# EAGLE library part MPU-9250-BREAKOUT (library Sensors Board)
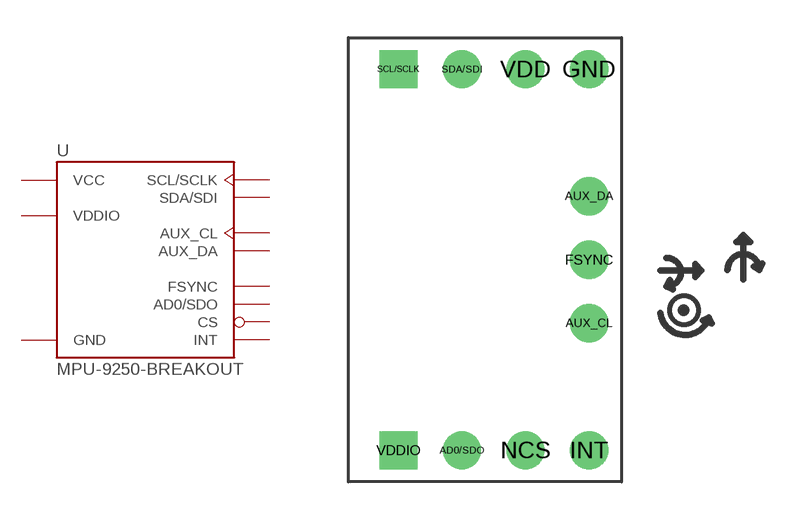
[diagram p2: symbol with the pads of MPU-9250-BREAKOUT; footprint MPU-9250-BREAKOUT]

Designator prefix -

## MPU-9250-BREAKOUT  [MPU-9250-BREAKOUT]
AD0/SDO  AD0/SDO  in
AUX_CL  AUX_CL  out
AUX_DA  AUX_DA
FSYNC  FSYNC  in
GND  GND  pwr
INT  INT  out
NCS  CS  in
SCL/SCLK  SCL/SCLK  in
SDA/SDI  SDA/SDI
VDD  VCC  pwr
VDDIO  VDDIO  pwr

## Footprint MPU-9250-BREAKOUT (pad centres in mm)
drill 1.016: AD0/SDO -0.533,-7.62; AUX_CL 4.547,-2.54; AUX_DA 4.547,2.54; FSYNC 4.547,0; GND 4.547,7.62; INT 4.547,-7.62; NCS 2.007,-7.62; SDA/SDI -0.533,7.62; VDD 2.007,7.62
drill 1.016 square: SCL/SCLK -3.073,7.62; VDDIO -3.073,-7.62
